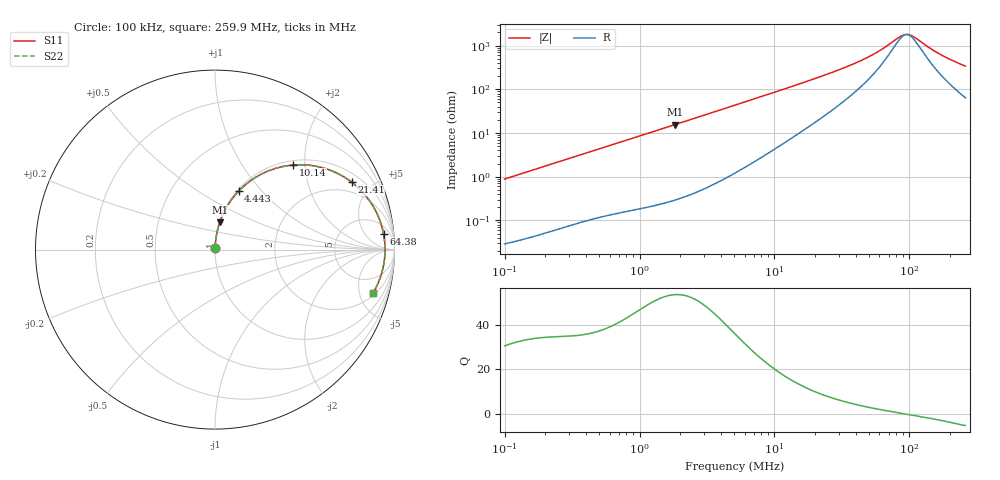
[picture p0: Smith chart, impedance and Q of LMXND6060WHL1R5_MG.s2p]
! LMXND6060WHL1R5_MG  S-PARAMETER MODEL  ( General Type )
! Model Generated by TAIYO YUDEN Corporation (https://www.yuden.co.jp/en/)
! Version 1.0
! TAIYO YUDEN Control No. 191025NI43SB-FBB
! Copyright(c) 2019 TAIYO YUDEN CO.,LTD. All Rights Reserved.
! Product Description (link to TY-COMPAS)
! https://ds.yuden.co.jp/TYCOMPAS/or/detail?pn=LMXND6060WHL1R5NMG&u=M
! Products Name : Inductors
! Characteristics :
!  Inductance : 1.5 uH , SRF(min) : 78 MHz , DC Resistance(max) : 0.0208 Ohm
!  Rated Current : Saturation :5100 mA , Temp Rise : 4200 mA (40 degC)
!  Case Size : 6.0 x 6.0 / 0.236 x 0.236 [mm/inch] , Thickness : 2.8 / 0.11 [mm/inch]
!  (Conditions: Temperature = 25 degC , DC Bias Current/Voltage = 0A / 0V)
! External Node Assignments :
!  1  o---GGG---o  2
! GND o---------o GND
! Frequency Range : 0.1MHz  -  259.929867MHz  [ 402 STEP ]
# MHz S RI R 50
! Freq[MHz].  S11 Real  S11 Imag  S21 Real  S21 Imag  S12 Real  S12 Imag  S22 Real  S22 Imag
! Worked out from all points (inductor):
!   401 points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, 100 kHz to 259.9 MHz, reference 50 ohm
!   read as one part in series: L = 1.41 uH near 104 kHz
!   highest Q = 53.3 at 1.834 MHz (marker M1), where L = 1.35 uH
!   self-resonance near 95.62 MHz
!   S11 on the Smith chart (normalised r, x): 100 kHz: 1.00, +0.02; 4.443 MHz: 1.02, +0.76; 10.14 MHz: 1.09, +1.74; 21.41 MHz: 1.41, +3.79; 64.38 MHz: 9, +15; 259.9 MHz: 2.28, -6.66
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0.1  0.000368 0.00885  0.9996 -0.00885  0.9996 -0.00885  0.000368 0.00885
0.37324  0.00196 0.0323  0.998 -0.0323  0.998 -0.0323  0.00196 0.0323
1.393082  0.0161 0.1165  0.9839 -0.1165  0.9839 -0.1165  0.0161 0.1165
1.834412  0.0265 0.1515  0.9735 -0.1515  0.9735 -0.1515  0.0265 0.1515
2.998647  0.0654 0.2371  0.9346 -0.2371  0.9346 -0.2371  0.0654 0.2371
4.442916  0.1313 0.3253  0.8687 -0.3253  0.8687 -0.3253  0.1313 0.3253
5.098332  0.1654 0.3579  0.8346 -0.3579  0.8346 -0.3579  0.1654 0.3579
6.982683  0.2693 0.426  0.7307 -0.426  0.7307 -0.426  0.2693 0.426
10.14444  0.4343 0.4711  0.5657 -0.4711  0.5657 -0.4711  0.4343 0.4711
13.62339  0.5763 0.4618  0.4237 -0.4618  0.4237 -0.4618  0.5763 0.4618
19.02902  0.7191 0.4046  0.2809 -0.4046  0.2809 -0.4046  0.7191 0.4046
21.41112  0.7608 0.3763  0.2392 -0.3763  0.2392 -0.3763  0.7608 0.3763
28.75388  0.8423 0.2971  0.1577 -0.2971  0.1577 -0.2971  0.8423 0.2971
40.16316  0.9002 0.2059  0.0998 -0.2059  0.0998 -0.2059  0.9002 0.2059
51.85739  0.926 0.1406  0.074 -0.1406  0.074 -0.1406  0.926 0.1406
64.37529  0.9389 0.0889  0.0611 -0.0889  0.0611 -0.0889  0.9389 0.0889
71.02397  0.9427 0.0664  0.0573 -0.0664  0.0573 -0.0664  0.9427 0.0664
88.1685  0.947 0.0179  0.053 -0.0179  0.053 -0.0179  0.947 0.0179
95.38103  0.9473 0.000538  0.0527 -0.000538  0.0527 -0.000538  0.9473 0.000538
101.1751  0.9472 -0.0125  0.0528 0.0125  0.0528 0.0125  0.9472 -0.0125
168.6705  0.9292 -0.1298  0.0708 0.1298  0.0708 0.1298  0.9292 -0.1298
259.9299  0.8811 -0.2416  0.1189 0.2416  0.1189 0.2416  0.8811 -0.2416
